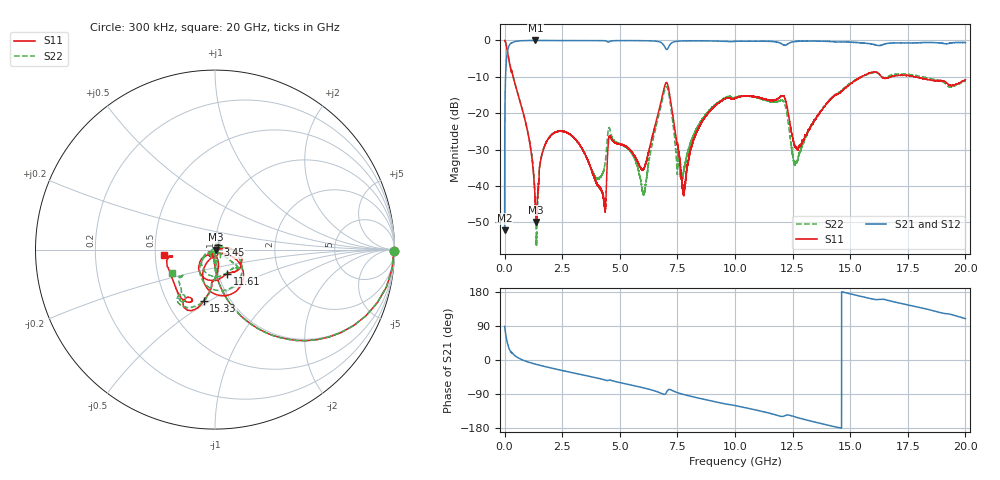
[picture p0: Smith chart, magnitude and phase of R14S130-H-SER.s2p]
!{R14S130}
!Johanson Technology Inc.
!www.johansontechnology.com
!Test Board Conditions:
!Substrate Type  RO4350B
!Substrate Thickness  20 mil
!Substrate Dk  3.66
!TL Type: GCPW
!TL Trace Width  36 mil
!TL Gap  12 mil
!Electrode orientation  Horizontal
!DUT TOPOLOGY	SERIES
!Mounting Pad LxW  26x36 mil
! Created Wed Nov 25 17:33:21 2020
! 2 Port Network Data from SP1.SP block
! freq  magS11  angS11  magS21  angS21  magS12  angS12  magS22  angS22
# khz S ma R 50
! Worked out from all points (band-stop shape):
!   20001 points, 300 kHz to 20 GHz, reference 50 ohm
!   highest |S21| = 0.00 dB at 1.338 GHz (marker M1); lowest = -52.2 dB at 300 kHz (marker M2)
!   |S21| within 3 dB of the highest: 122.5 MHz to end of sweep
!   lowest |S11| = -49.9 dB at 1.375 GHz (marker M3), VSWR 1.01, Z = 50.3 - j0.0323 ohm
!   |S11| at or under -10 dB: 370.3 MHz to 15.49 GHz (15.12 GHz wide, 191 % of centre); 16.36 GHz to 16.74 GHz (378.8 MHz wide, 2.29 % of centre); 17.84 GHz to end of sweep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
!   |S22| runs from -56.6 to 0.0 dB; largest |S21 - S12| = 0.021
!   S11 on the Smith chart (normalised r, x): 300 kHz: open; 3.45 GHz: 1.03, +0.05; 11.61 GHz: 1.10, -0.30; 15.33 GHz: 0.75, -0.47; 20 GHz: 0.55, -0.04
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300  0.9963 -0.3  0.002444 89.2  0.002475 90.0  0.996 -0.3
102300  0.7649 -40.9  0.641 49.1  0.6419 48.9  0.7659 -40.8
177300  0.5598 -57.2  0.8233 32.7  0.8255 32.5  0.5626 -57.1
1338300  0.005322 -64.3  0.9995 -10.9  0.9984 -10.9  0.005451 -119.2
1375300  0.003181 -5.8  0.9988 -11.5  0.9991 -11.5  0.001937 -159.3
1937300  0.04655 65.2  0.9972 -20.0  0.9972 -20.0  0.0463 72.6
3334300  0.03373 55.8  0.9975 -38.6  0.9976 -38.6  0.03365 43.8
3450300  0.02898 57.8  0.9983 -40.1  0.9966 -40.1  0.02868 38.7
4307300  0.006416 109.7  0.9922 -51.8  0.9932 -51.9  0.01656 -45.3
4594300  0.04712 -135.4  0.9766 -53.3  0.9768 -53.3  0.05538 -107.3
6034300  0.01712 -82.1  0.9924 -73.7  0.9922 -73.7  0.007564 118.9
6667300  0.09929 -22.4  0.9677 -84.8  0.966 -84.7  0.08726 -0.3
7080300  0.2456 -91.5  0.7718 -79.9  0.7711 -79.9  0.2157 -97.1
7772300  0.008293 -56.4  0.9863 -91.0  0.9863 -91.0  0.01582 -58.8
8537300  0.07359 6.0  0.9889 -102.2  0.9879 -102.2  0.07909 -35.6
1.00003e7  0.1598 -27.0  0.9721 -120.1  0.971 -120.1  0.164 -39.3
1.16133e7  0.1497 -63.5  0.9678 -142.3  0.9666 -142.3  0.1435 -49.8
1.26183e7  0.0337 -122.8  0.9684 -150.3  0.9703 -150.4  0.02121 -119.3
1.33343e7  0.06998 -75.0  0.9811 -161.9  0.9829 -161.8  0.069 -85.7
1.53333e7  0.2946 -102.5  0.9358 169.8  0.9409 169.6  0.2978 -103.1
1.66673e7  0.3071 -114.4  0.9166 157.0  0.9104 156.6  0.3234 -120.9
2e7  0.2884 -173.6  0.9353 109.3  0.9326 109.5  0.2759 -151.2
